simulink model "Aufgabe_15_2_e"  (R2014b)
settings: Solver=ode45  StartTime=0.0  StopTime=10.0  RelTol=1e-3

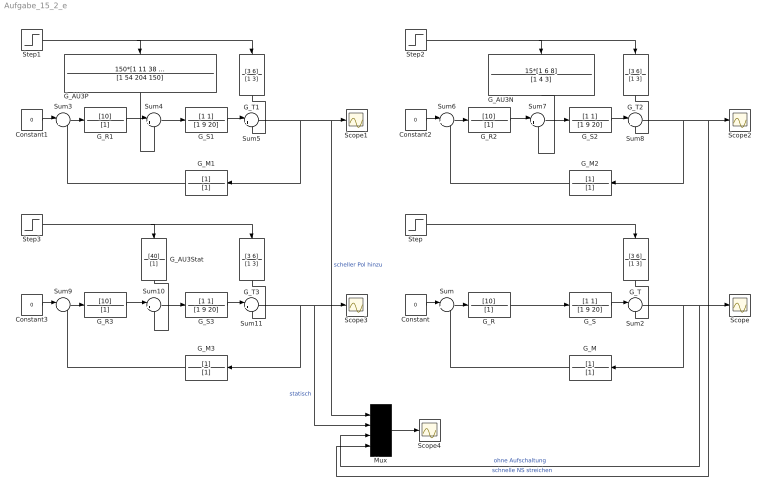
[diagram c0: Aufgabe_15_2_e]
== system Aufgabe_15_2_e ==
  Constant{,1..3} (4 alike) : Constant  Value=0
  G_AU3N : TransferFcn  Numerator=15*[1 6 8]  Denominator=[1 4 3]
  G_AU3P : TransferFcn  Numerator=150*[1 11 38 40]  Denominator=[1 54 204 150]
  G_AU3Stat : TransferFcn  Numerator=[40]  Denominator=[1]
  G_M{,1..3} (4 alike) : TransferFcn  Denominator=[1]
  G_R{,1..3} (4 alike) : TransferFcn  Numerator=[10]  Denominator=[1]
  G_S{,1..3} (4 alike) : TransferFcn  Numerator=[1 1]  Denominator=[1 9 20]
  G_T{,1..3} (4 alike) : TransferFcn  Numerator=[3 6]  Denominator=[1 3]
  Mux : Mux
  Scope{,1..4} (5 alike) : Scope
  Step{,1..3} (4 alike) : Step  SampleTime=0
  Sum{,3..4,6..7,9..10} (7 alike) : Sum  Inputs=|+-
  Sum{2,5,8,11} (4 alike) : Sum  Inputs=|++
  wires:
  Step/1 -> G_T/1
  Constant/1 -> Sum/1
  Sum/1 -> G_R/1
  G_M/1 -> Sum/2
  G_S/1 -> Sum2/1
  G_T/1 -> Sum2/2
  Sum2/1 -> G_M/1, Mux/3, Scope/1  "ohne Aufschaltung"
  G_R/1 -> G_S/1
  Step1/1 -> G_T1/1, G_AU3P/1
  G_R1/1 -> Sum4/1
  Constant1/1 -> Sum3/1
  Sum3/1 -> G_R1/1
  G_M1/1 -> Sum3/2
  G_S1/1 -> Sum5/1
  G_T1/1 -> Sum5/2
  Sum5/1 -> G_M1/1, Mux/1, Scope1/1  "scheller Pol hinzu"
  G_AU3P/1 -> Sum4/2
  Sum4/1 -> G_S1/1
  Step2/1 -> G_T2/1, G_AU3N/1
  G_R2/1 -> Sum7/1
  Constant2/1 -> Sum6/1
  Sum6/1 -> G_R2/1
  G_M2/1 -> Sum6/2
  G_S2/1 -> Sum8/1
  G_T2/1 -> Sum8/2
  Sum8/1 -> G_M2/1, Mux/4, Scope2/1  "schnelle NS streichen"
  G_AU3N/1 -> Sum7/2
  Sum7/1 -> G_S2/1
  Step3/1 -> G_T3/1, G_AU3Stat/1
  G_R3/1 -> Sum10/1
  Constant3/1 -> Sum9/1
  Sum9/1 -> G_R3/1
  G_M3/1 -> Sum9/2
  G_S3/1 -> Sum11/1
  G_T3/1 -> Sum11/2
  Sum11/1 -> G_M3/1, Mux/2, Scope3/1  "statisch"
  G_AU3Stat/1 -> Sum10/2
  Sum10/1 -> G_S3/1
  Mux/1 -> Scope4/1
